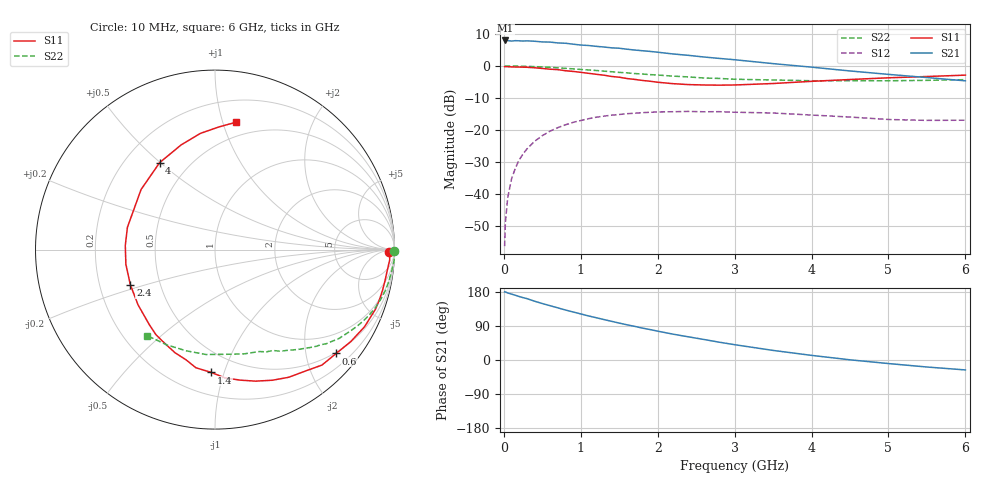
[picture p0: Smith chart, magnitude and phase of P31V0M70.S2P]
! SIEMENS Small Signal Semiconductors
! BFP181
! Si NPN RF Bipolar Junction Transistor in SOT143
! VCE = 1 V  IC = 0.7 mA
! Common Emitter S-Parameters:  March  1996
# GHz  S  MA  R  50
!  f  S11  S21  S12  S22
! GHz  MAG  ANG  MAG  ANG  MAG  ANG  MAG  ANG
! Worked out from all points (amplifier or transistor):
!   36 points, 10 MHz to 6 GHz, reference 50 ohm
!   highest |S21| = 8.0 dB at 20 MHz (marker M1)
!   |S21| within 3 dB of that: start of sweep to 1.7 GHz
!   unconditionally stable (mu >= 1): 3.301 GHz to end of sweep
!   at 250 MHz: K = 0.09, MSG = 17.7 dB, |S12| = -27.6 dB
!   at 1.4 GHz: K = 0.48, MSG = 10.6 dB, |S12| = -15.4 dB
!   at 6 GHz: K = 1.45, MAG = 2.2 dB, |S12| = -17.0 dB
!   S11 on the Smith chart (normalised r, x): 10 MHz: 57, -28; 600 MHz: 0.47, -2.63; 1.4 GHz: 0.35, -0.91; 2.4 GHz: 0.34, -0.18; 4 GHz: 0.34, +0.50; 6 GHz: 0.38, +1.10
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0.01  0.9719 -0.8  2.489 179.7  0.0015 85.2  0.9988 -0.3
0.02  0.9746 -1.5  2.51 179.5  0.0035 87.7  0.9976 -0.7
0.05  0.9748 -3.5  2.495 177.0  0.0086 90.7  0.9975 -1.7
0.1  0.9667 -6.9  2.456 173.9  0.017 84.5  1 -3.4
0.15  0.9629 -10.4  2.491 170.8  0.025 82.2  0.9949 -5.1
0.2  0.9607 -13.6  2.477 167.5  0.0339 80.8  0.9924 -6.8
0.3  0.9537 -20.4  2.476 162.0  0.05 76.0  0.9854 -10.1
0.4  0.9376 -27.3  2.439 155.1  0.066 71.1  0.9769 -13.4
0.6  0.8893 -40.6  2.367 143.4  0.0951 62.1  0.9511 -19.7
0.8  0.8423 -53.6  2.27 132.0  0.1196 53.7  0.9184 -25.4
1.1  0.7668 -72.9  2.092 116.3  0.1491 42.0  0.865 -33.2
1.4  0.6845 -91.8  1.923 102.1  0.1694 31.8  0.8121 -40.2
1.5  0.6668 -99.2  1.896 97.4  0.1735 29.0  0.7925 -42.0
1.8  0.5929 -118.1  1.733 84.2  0.1856 21.4  0.7473 -47.2
2.2  0.5277 -144.4  1.541 68.2  0.1918 11.7  0.6928 -54.1
2.4  0.5107 -157.4  1.467 61.1  0.194 7.3  0.6728 -57.3
3  0.5035 165.7  1.252 40.4  0.1884 -2.8  0.6192 -66.5
3.5  0.5308 140.9  1.088 25.3  0.1832 -8.9  0.603 -74.5
4  0.5743 122.5  0.958 12.2  0.1701 -13.4  0.5864 -84.1
4.5  0.6132 107.9  0.835 0.5  0.1583 -17.1  0.5868 -94.8
5.5  0.6833 88.3  0.658 -18.5  0.1404 -13.9  0.595 -116.9
6  0.7182 80.8  0.585 -26.2  0.1412 -11.4  0.6103 -128.2
